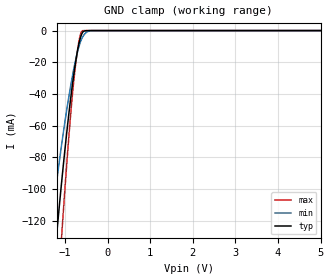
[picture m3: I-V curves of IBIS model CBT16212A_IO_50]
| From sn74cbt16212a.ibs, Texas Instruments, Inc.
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[Model]   CBT16212A_IO_50
Model_type  Terminator
| variable   typ   min   max
C_comp   5.41pF   4.23pF   9.95pF
| C_tri-state   5.41pF   4.23pF   9.95pF
[Temperature Range]   40   100   -40
| Ambient temperature   25   85   -40
[Voltage range]   5   4.5   5.5
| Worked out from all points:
|   GND clamp passes 1 mA (typ) near -0.58 V on its own axis
[GND Clamp]
| CBT16212A_IO_50
|   Voltage   I(typ)   I(min)   I(max)
-5V       -1.648A    -1.248A    -2.241A
-1.375V   -183.3mA   -134.3mA   -256.1mA
-1.33V    -169.2mA   -124.1mA   -235.9mA
-1.19V    -126.8mA   -93.99mA   -175mA
-1.07V    -92.98mA   -70.07mA   -126mA
-905mV    -51.26mA   -40.84mA   -65.13mA
-790mV    -26.81mA   -23.59mA   -30.49mA
-680mV    -9.042mA   -10.7mA    -7.752mA
-630mV    -3.778mA   -6.518mA   -1.653mA
-590mV    -1.22mA    -4.149mA   -82.86uA
-335mV    -398.2nA   -27.67uA   -3.517nA
5V        97.12pA    3.309nA    47.17pA
